FUNCTION_BLOCK Example14_DOcmdlb //4x3 flyways 1 xbot - DO set on cmdlb, DI as reset, read DO from PMC
VAR_INPUT
	Execute : BOOL;
END_VAR
VAR_OUTPUT
	Done : BOOL;
END_VAR
VAR_IN_OUT
	PM_Controller : PMControllerType;	// the planar motor controller to use
END_VAR
VAR
	PMC_XYMotion1 : PMC_XYMotion;
	DoID_array5 : ARRAY[0..4] OF USINT;
	xbotID_array5 : ARRAY[0..4] OF USINT;
	cmdlabel_array5 : ARRAY[0..4] OF UINT;
	type_array5 : ARRAY[0..4] OF USINT;
	PMC_ConfigDO2CmdLb1 : PMC_ConfigDO2CmdLb;
	PMC_XYMotion2 : PMC_XYMotion;
	first_read : BOOL;
	PMC_ReadDigitalSignalFromPMC1 : PMC_ReadDigitalSignalFromPMC;
	DI_ID_array22 : ARRAY[0..21] OF USINT;
	Rst_DO_ID_array22 : ARRAY[0..21] OF USINT;
	PMC_ConfigDI2Reset1 : PMC_ConfigDI2Reset;
	PMC_SendDigitalSignalToPMC1 : PMC_SendDigitalSignalToPMC;
	Delay1 : Delay;
	PMC_SendDigitalSignalToPMC2 : PMC_SendDigitalSignalToPMC;
	Delay2 : Delay;
	second_read : BOOL;
	PMC_ReadDigitalSignalFromPMC2 : PMC_ReadDigitalSignalFromPMC;
END_VAR

//4x3 flyways 1 xbot - DO set on cmdlb, DI as reset, read DO from PMC

//move xbot 1 to 60,60
PMC_XYMotion1(Execute := Execute,cmdLB := 1,XbotID := 1,Mode := 0,Type_ := 0,PosX := 0.06,PosY := 0.06,EndVel := 0,MaxVel := 1,MaxAcc := 10,PM_Controller := PM_Controller);

//config DO1 to set on a cmdlb (3)
DoID_array5[0] := 1;
xbotID_array5[0] := 1;
cmdlabel_array5[0] := 3;
type_array5[0] := 0;
PMC_ConfigDO2CmdLb1(Execute := PMC_XYMotion1.Done,nDO := 1,DoID := DoID_array5,XbotID := xbotID_array5,CmdLb := cmdlabel_array5,Type_ := type_array5,PM_Controller := PM_Controller);

//cmd label 3
PMC_XYMotion2(Execute := PMC_ConfigDO2CmdLb1.Done,cmdLB := 3,XbotID := 1,Mode := 0,Type_ := 0,PosX := 0.9,PosY := 0.06,EndVel := 0,MaxVel := 1,MaxAcc := 10,PM_Controller := PM_Controller);

//read DO 1 
PMC_ReadDigitalSignalFromPMC1(Enable := PMC_XYMotion2.Done,DiID := 1,PM_Controller := PM_Controller);
//only record the output of the first read once
IF(PMC_ReadDigitalSignalFromPMC1.Valid = TRUE AND PMC_ConfigDI2Reset1.Done = FALSE) THEN
	first_read := PMC_ReadDigitalSignalFromPMC1.Level;
END_IF;

//setup DI 1 as reset for DO 1
DI_ID_array22[0] := 1;
Rst_DO_ID_array22[0] := 1;
PMC_ConfigDI2Reset1(Execute := PMC_ReadDigitalSignalFromPMC1.Valid,nDI := 1,DiID := DI_ID_array22,RstDoID := Rst_DO_ID_array22,PM_Controller := PM_Controller);

//set DI 1 to 0
PMC_SendDigitalSignalToPMC1(Enable := PMC_ConfigDI2Reset1.Done,DoID := 1,Level := FALSE,PM_Controller := PM_Controller);

Delay1(Execute := PMC_SendDigitalSignalToPMC1.Valid,Cycles := 1);

//set DI 1 to 1
PMC_SendDigitalSignalToPMC2(Enable := Delay1.Done,DoID := 1,Level := TRUE,PM_Controller := PM_Controller);

Delay2(Execute := PMC_SendDigitalSignalToPMC2.Valid,Cycles := 1);

//read DO1
PMC_ReadDigitalSignalFromPMC2(Enable := Delay2.Done,DiID := 1,Level => second_read,PM_Controller := PM_Controller);

Done := PMC_ReadDigitalSignalFromPMC2.Valid;

END_FUNCTION_BLOCK
